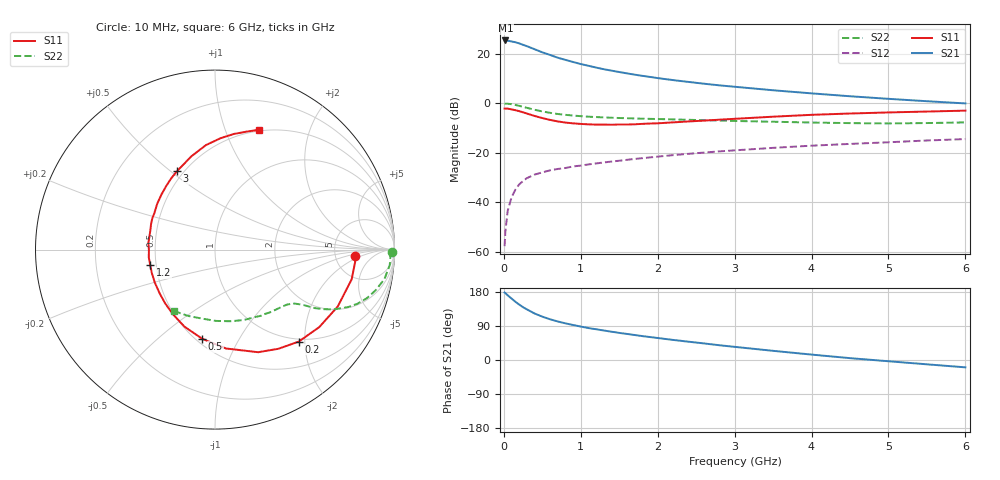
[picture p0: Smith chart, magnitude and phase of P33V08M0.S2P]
! SIEMENS Small Signal Semiconductors
! BFP181
! Si NPN RF Bipolar Junction Transistor in SOT143
! VCE = 3 V  IC = 8 mA
! Common Emitter S-Parameters:  March  1996
# GHz  S  MA  R  50
!  f  S11  S21  S12  S22
! GHz  MAG  ANG  MAG  ANG  MAG  ANG  MAG  ANG
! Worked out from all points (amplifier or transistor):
!   36 points, 10 MHz to 6 GHz, reference 50 ohm
!   highest |S21| = 25.4 dB at 20 MHz (marker M1)
!   |S21| within 3 dB of that: start of sweep to 355.6 MHz
!   unconditionally stable (mu >= 1): 1.302 GHz to end of sweep
!   at 250 MHz: K = 0.30, MSG = 27.5 dB, |S12| = -31.4 dB
!   at 1.4 GHz: K = 1.03, MAG = 17.3 dB, |S12| = -23.5 dB
!   at 6 GHz: K = 1.01, MAG = 6.5 dB, |S12| = -14.5 dB
!   S11 on the Smith chart (normalised r, x): 10 MHz: 7.91, -1.44; 200 MHz: 0.95, -1.87; 500 MHz: 0.54, -0.71; 1.2 GHz: 0.46, -0.09; 3 GHz: 0.46, +0.53; 6 GHz: 0.49, +1.31
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0.01  0.782 -2.6  18.52 178.0  0.0013 85.2  0.9849 -0.8
0.02  0.7837 -5.2  18.56 176.6  0.0026 91.3  0.9778 -1.9
0.05  0.7794 -12.2  18.37 170.8  0.0067 84.4  0.9777 -5.0
0.1  0.754 -24.8  17.71 162.2  0.0126 77.2  0.9586 -9.8
0.15  0.7239 -36.6  17.08 153.7  0.018 70.9  0.9243 -14.1
0.2  0.693 -47.7  16.2 146.2  0.023 66.6  0.8877 -17.8
0.25  0.6558 -57.4  15.14 139.3  0.0269 63.2  0.8478 -20.9
0.3  0.6202 -67.2  14.23 133.5  0.0308 60.1  0.8086 -23.3
0.4  0.5542 -83.7  12.33 122.7  0.0363 54.5  0.7395 -26.8
0.5  0.5021 -98.1  10.68 114.4  0.0402 51.1  0.6842 -29.0
0.6  0.4621 -111.5  9.467 107.5  0.0442 49.3  0.6413 -30.5
0.7  0.4297 -123.1  8.328 101.7  0.0471 47.8  0.6081 -31.3
0.9  0.393 -141.7  6.82 92.4  0.053 46.6  0.5647 -32.7
1.1  0.3755 -159.6  5.715 84.3  0.0582 46.0  0.536 -34.1
1.2  0.3708 -166.8  5.262 81.1  0.0609 45.8  0.5263 -35.0
1.7  0.3761 163.2  3.784 66.0  0.0751 45.3  0.4936 -39.8
2.2  0.4115 141.4  2.938 53.0  0.0896 43.8  0.4719 -46.1
3  0.4854 115.9  2.154 34.7  0.1119 39.5  0.4392 -58.5
3.5  0.5357 104.3  1.831 24.2  0.1258 36.3  0.4238 -67.8
4.5  0.6212 87.2  1.386 4.9  0.1511 29.0  0.3974 -89.2
5.5  0.6805 75.0  1.1 -11.4  0.1772 22.3  0.3986 -111.9
6  0.7099 70.0  0.993 -19.4  0.1892 18.3  0.4109 -123.5
